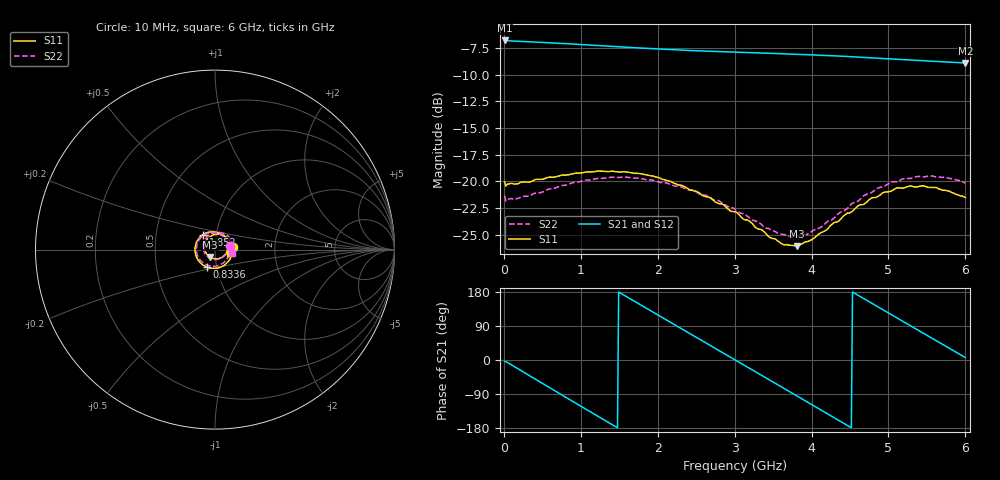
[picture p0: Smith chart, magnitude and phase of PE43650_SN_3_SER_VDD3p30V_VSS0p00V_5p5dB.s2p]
!Keysight Technologies,N5245B,MY57181451,A.13.50.07
!Date: Tuesday, May 07, 2019 07:59:55
!Correction: S11(Full 2 Port(1,2))
!S21(Full 2 Port(1,2))
!S12(Full 2 Port(1,2))
!S22(Full 2 Port(1,2))
!S2P File: Measurements: S11, S21, S12, S22:
# Hz S  dB  R 50
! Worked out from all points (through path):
!   401 points, 10 MHz to 6 GHz, reference 50 ohm
!   highest |S21| = -6.81 dB at 10 MHz (marker M1); lowest = -8.9 dB at 6 GHz (marker M2)
!   group delay of S21, straight-line fit = 329 ps
!   lowest |S11| = -26.1 dB at 3.814 GHz (marker M3), VSWR 1.10, Z = 47.1 - j3.88 ohm
!   |S11| at or under -10 dB: start of sweep to end of sweep
!   |S22| runs from -25.2 to -19.5 dB; largest |S21 - S12| = 0.0033
!   S11 on the Smith chart (normalised r, x): 10 MHz: 1.22, +0.04; 833.6 MHz: 0.89, -0.18; 1.852 GHz: 0.86, +0.15; 6 GHz: 1.18, -0.05
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1e7  -20.06 9.7  -6.81 -3.4  -6.85 -3.3  -21.36 13.2
2.34625e8  -20.08 -34.5  -6.90 -29.3  -6.95 -29.3  -21.45 -34.8
4.74225e8  -19.83 -68.1  -6.98 -58.4  -7.04 -58.4  -21.08 -68.8
8.33625e8  -19.39 -115.7  -7.12 -101.8  -7.17 -101.8  -20.28 -116.1
1.013325e9  -19.21 -138.1  -7.20 -123.4  -7.25 -123.4  -19.97 -137.8
1.432625e9  -19.07 173.7  -7.37 -173.5  -7.43 -173.5  -19.62 175.6
1.851925e9  -19.40 128.8  -7.55 136.6  -7.61 136.6  -19.86 132.2
2.01665e9  -19.67 111.8  -7.61 117.1  -7.66 117.2  -20.06 115.9
2.241275e9  -20.26 88.3  -7.69 90.6  -7.75 90.6  -20.45 93.2
2.4659e9  -20.88 64.3  -7.76 64.1  -7.82 64.1  -20.88 70.5
2.750425e9  -21.96 34.0  -7.84 30.5  -7.90 30.6  -21.77 40.0
3.005e9  -22.86 2.7  -7.90 0.5  -7.96 0.5  -22.62 10.9
3.45425e9  -25.25 -61.0  -8.01 -52.7  -8.06 -52.6  -24.47 -51.8
3.81365e9  -26.08 -124.3  -8.11 -95.3  -8.16 -95.3  -25.15 -111.3
4.008325e9  -25.44 -158.4  -8.16 -118.4  -8.21 -118.4  -24.68 -144.5
4.2629e9  -24.06 161.5  -8.24 -148.6  -8.30 -148.6  -23.62 175.5
4.5025e9  -22.93 128.6  -8.33 -177.1  -8.39 -176.9  -22.25 141.5
4.7421e9  -21.77 99.0  -8.43 154.5  -8.48 154.7  -21.15 112.7
5.01165e9  -20.97 70.2  -8.53 122.7  -8.58 122.9  -20.16 81.9
5.4609e9  -20.44 27.3  -8.71 69.8  -8.76 69.9  -19.59 37.0
5.745425e9  -20.87 4.1  -8.83 36.3  -8.87 36.4  -19.63 11.1
6e9  -21.51 -13.8  -8.92 6.4  -8.97 6.5  -20.17 -10.4
